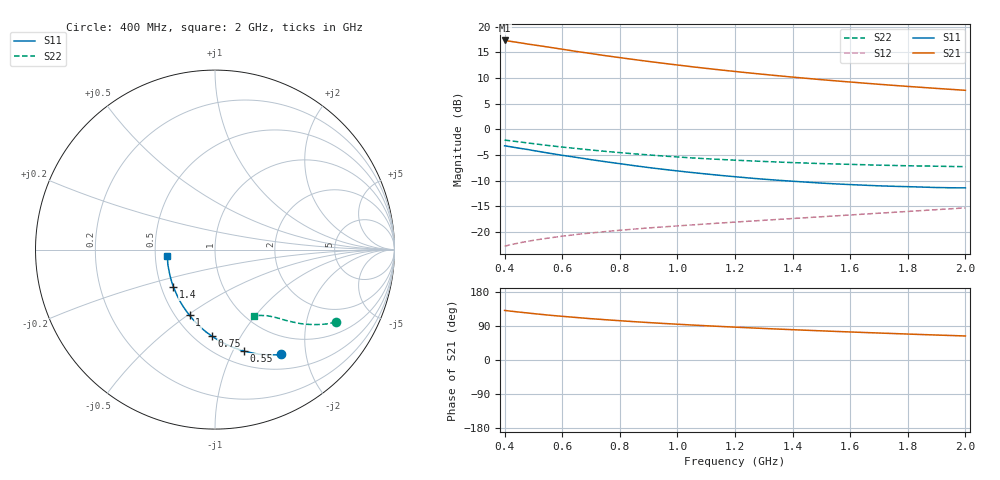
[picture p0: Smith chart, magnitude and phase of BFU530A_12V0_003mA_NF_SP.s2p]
! Filename:  P:\Prog\Test\Noise\ATS_data\Testdata_Net\06 Compressed Noise after Statistics\BFU530A_APG2013_33_A05_12p0V_003mA_NF_CM01_D.sf
! Date/Time: Tue 16/Apr/2013 15:10:59
! BFU530A_APG2013_33_A05_12p0V_1to25mA_NF_CM01_Bias3_R.sf
! Noise Parameter Data File
! BFU530A_APG2013_33_A05_12p0V_1to25mA_NF_CM01
! Date/time: Fri Apr 12 17:55:00 2013
! VAR V_out= 12.001000
! VAR I_out= 2.995000
! VAR V_in= 0.800000
! VAR I_in= 0.024505
! Device data file deembeded for feedlines and parallel
! Original file: \06 Compressed Noise after Statistics\BFU530A_APG2013_33_A05_12p0V_003mA_NF_CM01_R.sf
! Feed-files: PR017V01_150413_Feed1.s2p, PR017V01_150413_Feed2.s2p
! Parallel-file: PR017V01_150413_Par.s2p
# MHz S MA R 50
!  Freq-MHz  S11-mag  S11-arg  S21-mag  S21-arg  S12-mag  S12-arg  S22-mag  S22-arg
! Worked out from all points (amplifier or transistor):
!   37 points, 400 MHz to 2 GHz, reference 50 ohm
!   highest |S21| = 17.3 dB at 400 MHz (marker M1)
!   |S21| within 3 dB of that: start of sweep to 755.1 MHz
!   unconditionally stable (mu >= 1): 1.879 GHz to end of sweep
!   at 500 MHz: K = 0.44, MSG = 19.0 dB, |S12| = -21.6 dB
!   at 1.1 GHz: K = 0.80, MSG = 15.2 dB, |S12| = -18.5 dB
!   at 2 GHz: K = 1.01, MAG = 10.8 dB, |S12| = -15.3 dB
!   lowest NFmin = 0.56 dB at 420 MHz
!   S11 on the Smith chart (normalised r, x): 400 MHz: 0.71, -1.57; 550 MHz: 0.64, -1.10; 750 MHz: 0.61, -0.76; 1 GHz: 0.59, -0.51; 1.4 GHz: 0.58, -0.27; 2 GHz: 0.58, -0.04
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400  0.6896 -57.9  7.314 130.9  0.07266 60.5  0.784 -30.9
420  0.6755 -60.3  7.178 129.0  0.07495 59.7  0.7714 -31.9
440  0.6609 -62.5  7.039 127.3  0.07704 58.9  0.7592 -32.8
480  0.6347 -66.8  6.75 124.1  0.08097 57.6  0.735 -34.4
550  0.587 -74.2  6.319 118.6  0.08696 55.6  0.695 -36.9
600  0.5573 -79.0  6.01 115.2  0.09083 54.6  0.6705 -38.4
650  0.5315 -83.4  5.713 112.1  0.09452 53.7  0.6488 -39.8
700  0.5056 -87.9  5.457 109.0  0.0977 53.0  0.6277 -41.0
750  0.4829 -92.0  5.201 106.3  0.1008 52.5  0.6087 -42.0
800  0.4619 -96.1  4.979 103.7  0.1038 52.1  0.5918 -43.0
850  0.4419 -100.1  4.767 101.1  0.1066 51.8  0.5758 -43.9
900  0.4235 -104.0  4.571 98.8  0.1094 51.6  0.5624 -44.7
950  0.4073 -107.6  4.39 96.5  0.1119 51.6  0.5486 -45.5
1000  0.3926 -111.2  4.22 94.4  0.1144 51.6  0.5371 -46.2
1100  0.3667 -118.2  3.913 90.4  0.1195 51.8  0.5162 -47.5
1200  0.3448 -125.0  3.65 86.7  0.1246 52.1  0.4995 -48.8
1300  0.3261 -131.4  3.42 83.2  0.1298 52.5  0.4855 -50.1
1400  0.3116 -138.0  3.217 80.0  0.135 53.1  0.4731 -51.3
1500  0.2989 -144.3  3.037 76.9  0.1405 53.6  0.4629 -52.6
1650  0.285 -153.2  2.808 72.6  0.1492 54.5  0.451 -54.5
1750  0.2782 -159.0  2.673 69.8  0.1552 55.1  0.4439 -55.8
2000  0.2684 -172.5  2.393 63.4  0.1715 56.4  0.432 -59.4
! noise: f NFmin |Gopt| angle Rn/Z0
400  0.628  0.346  20.55  0.1611
460  0.6039  0.3278  28.61  0.1514
600  0.6752  0.3477  31.31  0.1695
800  0.6718  0.3225  48.71  0.137
1000  0.7015  0.3047  63.83  0.1254
1200  0.7534  0.3007  77.56  0.1192
1400  0.7842  0.2899  90.64  0.1086
1600  0.7837  0.2824  108.8  0.0947
1800  0.751  0.2958  127.9  0.0782
2000  0.8133  0.2826  137.1  0.0778
